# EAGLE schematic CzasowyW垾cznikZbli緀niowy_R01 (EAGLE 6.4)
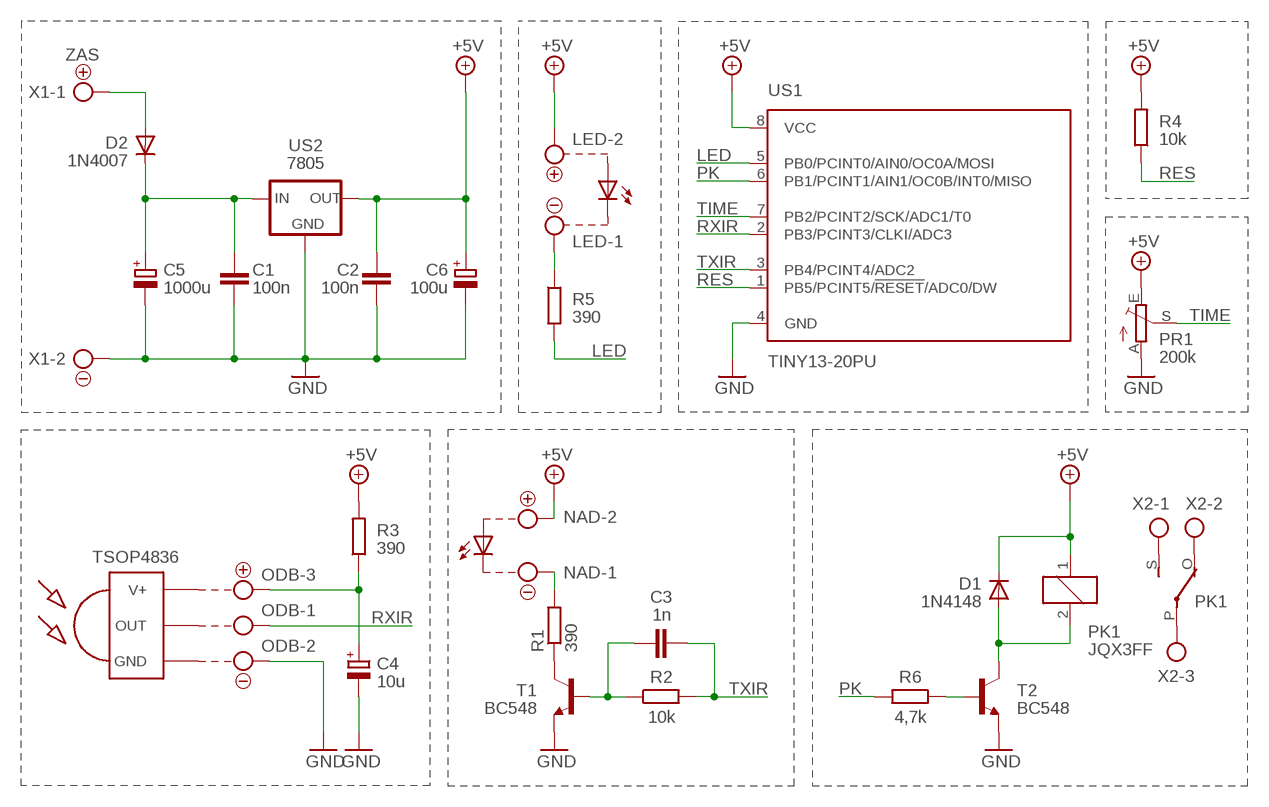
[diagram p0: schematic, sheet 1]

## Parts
C1  100n  C-EU050-025X075  [C050-025X075]
C2  100n  C-EU050-025X075  [C050-025X075]
C3  1n  C-EU050-025X075  [C050-025X075]
C4  10u  CPOL-EUE2.5-6  [E2,5-6]
C5  1000u  CPOL-EUE3.5-10  [E3,5-10]
C6  100u  CPOL-EUE3.5-8  [E3,5-8]
D1  1N4148  1N4148DO35-7  [DO35-7]
D2  1N4007  1N40047.62  [DO41-7.6]
LED  AK550/2  [AK550/2]
LED1  LED5MM  [LED5MM]
LED2  LED5MM  [LED5MM]
NAD  AK550/2  [AK550/2]
ODB  AK550/3  [AK550/3]
PK1  JQX3FF  G5LE  [G5LE]
PR1  200k  TRIM_EU-CA6V  [CA6V]
R1  390  R-EU_0207/7  [0207/7]
R2  10k  R-EU_0207/7  [0207/7]
R3  390  R-EU_0207/7  [0207/7]
R4  10k  R-EU_0207/7  [0207/7]
R5  390  R-EU_0207/7  [0207/7]
R6  4,7k  R-EU_0207/7  [0207/7]
T1  BC548  [TO92-EBC]
T2  BC548  [TO92-EBC]
U$1  TSOP4836  [TSOP18XX]
U$2  +  [+]
U$3  -  [-]
U$4  +  [+]
U$5  -  [-]
U$6  +  [+]
U$7  -  [-]
U$8  +  [+]
U$9  -  [-]
US1  TINY13-20PU  [DIL08]
US2  7805  78XXLNO_HOLE  [78XXL_H]
X1  ZAS  AK500/2  [AK500/2]
X2  NC COM NO  AK500/3  [AK500/3]

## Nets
+5V: C2.2 C6.+ D1.C LED.2 NAD.2 PK1.1 PR1.E R3.2 R4.2 US1.8(VCC) US2.OUT
GND: C1.1 C2.1 C4.- C5.- C6.- ODB.2 PR1.A T1.E T2.E US1.4(GND) US2.GND X1.2
LED: R5.2 US1.5(PB0/PCINT0/AIN0/OC0A/MOSI)
N$1: D1.A PK1.2 T2.C
N$3: R6.1 T2.B
N$4: PK1.S(2:S) X2.1
N$5: PK1.P(2:P) X2.3
N$6: PK1.O(2:O) X2.2
N$7: NAD.1 R1.2
N$8: R1.1 T1.C
N$9: D2.A X1.1
N$12: C1.2 C5.+ D2.C US2.IN
N$14: C3.2 R2.1 T1.B
N$19: C4.+ ODB.3 R3.1
N$22: LED.1 R5.1
PK: R6.2 US1.6(PB1/PCINT1/AIN1/OC0B/INT0/MISO)
RES: R4.1 US1.1(PB5/PCINT5/!RESET!/ADC0/DW)
RXIR: ODB.1 US1.2(PB3/PCINT3/CLKI/ADC3)
TIME: PR1.S US1.7(PB2/PCINT2/SCK/ADC1/T0)
TXIR: C3.1 R2.2 US1.3(PB4/PCINT4/ADC2)
Unconnected: LED1.A LED1.K(C) LED2.A LED2.K(C) U$1.GND U$1.OUT U$1.VCC(V+)

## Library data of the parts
C1-C3 = rcl:C-EU: CAPACITOR, European symbol
C4-C6 = rcl:CPOL-EU: POLARIZED CAPACITOR, European symbol
D1 = diode:1N4148: DIODE
D2 = diode:1N4004: DIODE
LED NAD = con-ptr500+:AK550/2: CONNECTOR
LED1 LED2 = led:LED: LED
ODB = con-ptr500+:AK550/3: CONNECTOR
PK1 = relay:G5LE: RELAY 1 x switch, 10 A/120 V AC, 8 A/30 V DC, Omron; OC_FARNELL: unknown; OC_NEWARK: unknown
PR1 = pot:TRIM_EU-: POTENTIOMETER
R1-R6 = rcl:R-EU_: RESISTOR, European symbol
T1 T2 = transistor-npn:BC548*: NPN Transistor
U$1 = tsop-1:TSOP4836: IR Receiver and Demodulator
U$2 U$4 U$6 U$8 = symbole:+
U$3 U$5 U$7 U$9 = symbole:-
US1 = atmel:TINY13: 8-bit AVR Microcontroller with 1K Bytes In-System Programmable Flash Source: http://www.atmel.com/dyn/resources/prod_documents/2535S.pdf; MPN: ATTINY13-20PU; OC_FARNELL: 9171550; OC_NEWARK: 96K6521
US2 = v-reg:78XXL: VOLTAGE REGULATOR
X1 = con-ptr500:AK500/2: CONNECTOR; OC_FARNELL: unknown; OC_NEWARK: unknown
X2 = con-ptr500:AK500/3: CONNECTOR; OC_FARNELL: unknown; OC_NEWARK: unknown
